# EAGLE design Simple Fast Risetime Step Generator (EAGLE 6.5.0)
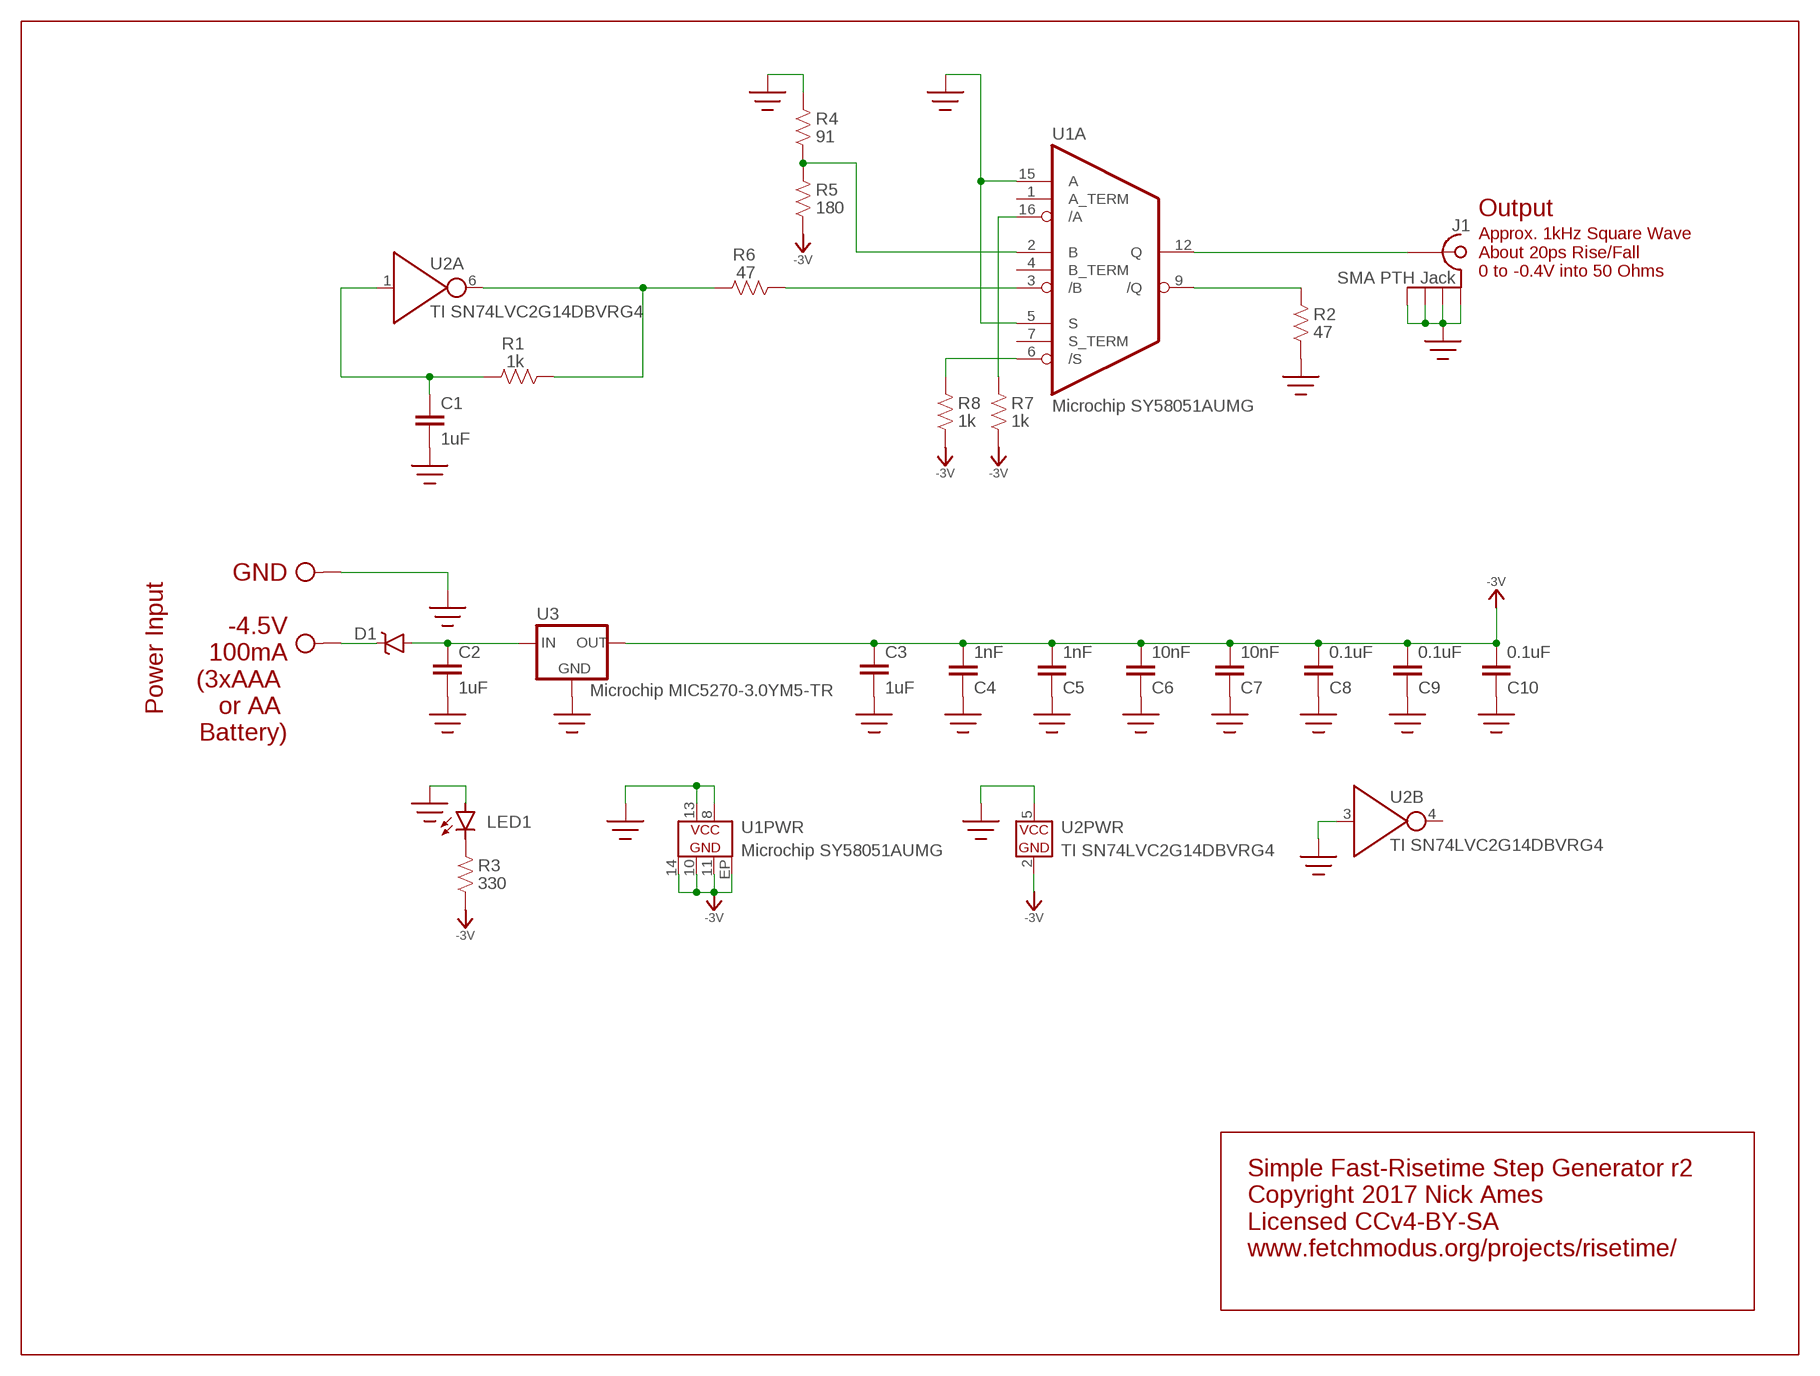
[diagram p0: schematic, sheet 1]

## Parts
C1  1uF  CAP402  [0402]
C2  1uF  CAP402  [0402]
C3  1uF  CAP402  [0402]
C4  1nF  CAP201  [0201]
C5  1nF  CAP201  [0201]
C6  10nF  CAP402  [0402]
C7  10nF  CAP402  [0402]
C8  0.1uF  CAP402  [0402]
C9  0.1uF  CAP402  [0402]
C10  0.1uF  CAP402  [0402]
D1  DIODE-SCHOTTKYSOD-523  [SOD-523]
J1  SMA PTH Jack  COAX-4GNDSMA-PTH  [CON-SMA-PTH]
LED1  LED0603  [LED-0603]
R1  1k  RESISTOR402  [0402@1]
R2  47  RESISTOR402  [0402@1]
R3  330  RESISTOR402  [0402@1]
R4  91  RESISTOR402  [0402@1]
R5  180  RESISTOR402  [0402@1]
R6  47  RESISTOR402  [0402@1]
R7  1k  RESISTOR402  [0402@1]
R8  1k  RESISTOR402  [0402@1]
TP1  TESTPOINTPTH  [TESTPOINT-1-PTH]
TP2  TESTPOINTPTH  [TESTPOINT-1-PTH]
U1  Microchip SY58051AUMG  SY58051AUMG  [QFN-16-3X3-MICREL]
U2  TI SN74LVC2G14DBVRG4  74LVC2G14  [SOT-23-6]
U3  Microchip MIC5270-3.0YM5-TR  V_REGSOT23-5-MIC5270  [SOT23-5]

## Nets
-3V: C3.1 C4.P$2 C5.P$2 C6.2 C7.2 C8.2 C9.2 C10.2 R3.1 R5.1 R7.1 R8.1 U1.10(PWR:V-) U1.11(PWR:V-1) U1.14(PWR:V-2) U1.EP(PWR:V-3) U2.2(PWR:V-) U3.4(OUT)
GND: C1.2 C2.2 C3.2 C4.P$1 C5.P$1 C6.1 C7.1 C8.1 C9.1 C10.1 J1.G1 J1.G2 J1.G3 J1.G4 LED1.A R2.1 R4.2 TP1.1 U1.5(A:S) U1.8(PWR:V+) U1.13(PWR:V+1) U1.15(A:A) U2.3(B:IN) U2.5(PWR:V+) U3.2(GND)
N$1: R6.1 U1.3(A:/B)
N$2: C1.1 R1.2 U2.1(A:IN)
N$3: R1.1 R6.2 U2.6(A:OUT)
N$4: D1.C TP2.1
N$5: R8.2 U1.6(A:/S)
N$6: C2.1 D1.A U3.5(IN)
N$7: J1.SIG(SIGNAL) U1.12(A:Q)
N$8: R2.2 U1.9(A:/Q)
N$9: LED1.C R3.2
N$10: R4.1 R5.2 U1.2(A:B)
N$13: R7.2 U1.16(A:/A)
Unconnected: U1.1(A:A_TERM) U1.4(A:B_TERM) U1.7(A:S_TERM) U2.4(B:OUT)

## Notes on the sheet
- Output
- Approx. 1kHz Square Wave
  About 20ps Rise/Fall
  0 to -0.4V into 50 Ohms
- GND
- -4.5V
  100mA
  (3xAAA 
  or AA 
  Battery)
- Power Input
- Simple Fast-Risetime Step Generator r2
  Copyright 2017 Nick Ames
  Licensed CCv4-BY-SA
  www.fetchmodus.org/projects/risetime/

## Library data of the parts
C1-C10 = NA-lib:CAP: Capacitor
D1 = NA-lib:DIODE-SCHOTTKY
J1 = NA-lib:COAX-4GND
LED1 = NA-lib:LED: LEDs
R1-R8 = NA-lib:RESISTOR: Resistor
TP1 TP2 = NA-lib:TESTPOINT
U1 = NA-lib:SY58051AUMG
U2 = NA-lib:74LVC2G14
U3 = NA-lib:V_REG

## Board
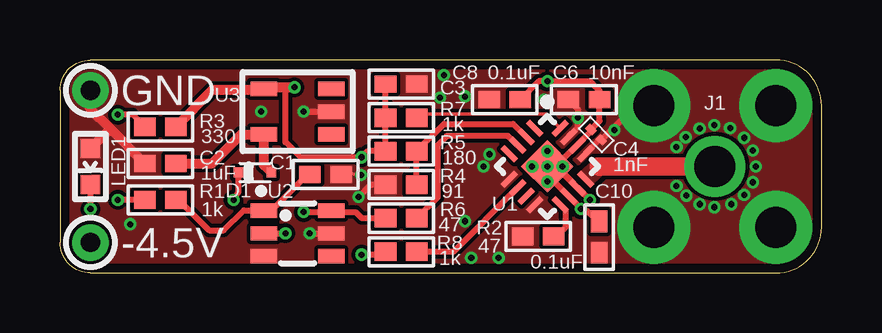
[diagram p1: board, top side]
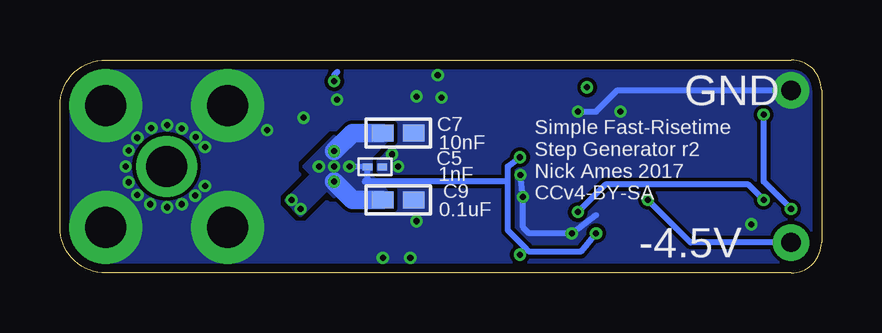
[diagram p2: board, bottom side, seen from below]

Size 31.75 x 8.89 mm. Coordinates in mm from the lower left corner, seen from the top.
Outline: 1.27,0 29.84,0 arc90 31.75,1.91 31.75,6.99 arc90 29.84,8.89 1.27,8.89 arc90 0,7.62 0,1.27 arc90 1.27,0
Copper layers (1*16): Top 0.0356mm / dielectric 1.5011mm / Bottom 0.0356mm
Design rules "LaenPCBOrder-tented_vias": minimum track width 6mil, minimum drill 10mil, track to track 6mil, track to pad 6mil, pad to pad 6mil, via to via 6mil, smd to smd 6mil, copper to edge 15mil, drill to drill 6mil, minimum pad ring 5mil, minimum via ring 5mil, stop-mask expansion 3mil, vias tented up to drill 25mil, thermal gap 10mil

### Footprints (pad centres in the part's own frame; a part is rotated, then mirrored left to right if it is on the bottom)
0402 = smd 0.9 x 0.7: 1 -0.65,0; 2 0.65,0
0201 = smd 0.406 x 0.279: P$1 -0.305,0; P$2 0.305,0
SOD-523 = smd 0.406 x 0.406: A 0.686,0; C -0.686,0
CON-SMA-PTH = drill 1.702 pad 3.048: G1 -2.54,2.54; G2 2.54,2.54; G3 -2.54,-2.54; G4 2.54,-2.54 | drill 1.702 pad 2.54: SIG 0,0
LED-0603 = smd 0.8 x 0.8: A -0.75,0; C 0.75,0
0402@1 = smd 0.9 x 0.762: 1 -0.65,0; 2 0.65,0
TESTPOINT-1-PTH = drill 0.8 pad 1.524: 1 0,0
QFN-16-3X3-MICREL = smd 0.8 x 0.23: 1 -1.5,0.75; 2 -1.5,0.25; 3 -1.5,-0.25; 4 -1.5,-0.75; 9 1.5,-0.75; 10 1.5,-0.25; 11 1.5,0.25; 12 1.5,0.75 | smd 0.23 x 0.8: 5 -0.75,-1.5; 6 -0.25,-1.5; 7 0.25,-1.5; 8 0.75,-1.5; 13 0.75,1.5; 14 0.25,1.5; 15 -0.25,1.5; 16 -0.75,1.5 | smd 1.55 x 1.55: EP 0,0
SOT-23-6 = smd 1.1 x 0.6: 1 -1.4,0.95; 2 -1.4,0; 3 -1.4,-0.95; 4 1.4,-0.95; 5 1.4,0; 6 1.4,0.95
SOT23-5 = smd 0.6 x 1.1: 1 -0.95,-1.4; 2 0,-1.4; 3 0.95,-1.4; 4 0.95,1.4; 5 -0.95,1.4

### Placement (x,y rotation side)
C1  11.07,4.11 0 top
C2  4.19,4.57 180 top
C3  14.22,7.87 0 top
C4  22.35,5.77 135 top
C5  18.62,4.42 180 bottom
C6  21.84,7.24 0 top
C7  17.65,5.84 180 bottom
C8  18.54,7.24 0 top
C9  17.65,3.05 180 bottom
C10  22.48,1.5 90 top
D1  8.13,4.19 0 top
J1  27.3,4.45 0 top
LED1  1.27,4.45 270 top
R1  4.19,3.05 0 top
R2  19.94,1.52 0 top
R3  4.19,6.1 180 top
R4  14.22,3.68 180 top
R5  14.22,5.08 0 top
R6  14.22,2.29 180 top
R7  14.22,6.48 0 top
R8  14.22,0.89 0 top
TP1  1.27,7.62 0 top
TP2  1.27,1.27 0 top
U1  20.32,4.45 315 top
U2  9.91,1.65 0 top
U3  9.91,6.73 90 top

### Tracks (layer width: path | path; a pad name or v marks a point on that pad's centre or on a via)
-3V  (via drill 0.25 pad 0.51)
  Top 0.254: 20.77,4.38 20.7,4.32 20.8,4.32 U1.11 21.59,3.56 v22.1,3.05 20.75,4.39 20.8,4.45 21.01,4.45 | 20.77,4.38 20.83,4.45 v20.95,4.45 | v20.32,3.81 20.32,4.06 20.35,4.06 U1.10 21.72,2.69 v21.72,2.67 21.86,2.67 C10.2 | 20.77,4.38 20.77,4.54 U1.14 22.14,5.91 C4.P$2 22.49,6.34 C6.2 22.49,7.61 22.1,8 v20.32,8 19.95,8 C8.2 | U2.2 v9.4,1.65 | 9.4,7.75 9.4,5.46 10.03,4.83 v12.57,4.83 12.83,5.08 R5.1 R7.1 C3.1 | R8.1 13.45,0.76 v12.57,0.76
  Top 0.406: R3.1 6.35,7.62 8.45,7.62 U3.4 8.57,7.75 9.4,7.75 v9.78,7.75
  Bottom 0.254: v19.68,4.45 C5.P$2 18.92,3.94 19.05,3.81 13.08,3.81 | v9.4,1.65 10.03,0.89 12.19,0.89 12.38,1.08 | 12.38,1.08 13.08,1.78 13.08,3.81 | 13.08,3.81 13.08,4.45 v12.57,4.83 | 20.19,8.38 20.32,8.26 v20.32,8 | v12.57,0.76 12.38,0.95 12.38,1.08
  Bottom 0.762: C7.2 19.56,5.84 v20.32,5.08 | C9.2 19.56,3.05 v20.32,3.81
  other vias: 20.32,4.45
  pour Bottom (no thermals): 19.05,4.45 20.32,5.71 21.59,4.45 20.32,3.17
  pour Bottom (no thermals): 20.68,3.43 21.72,2.39 22.35,3.02 21.29,4.09 20.75,3.56
  pour Bottom (no thermals): 18.72,4.09 18.72,4.83 18.08,5.46 19.43,5.46 19.74,5.16 19.74,3.73 19.43,3.43 18.08,3.43 18.08,3.45
GND  (via drill 0.25 pad 0.51)
  Top 0.152: C1.2 11.73,4.19 v12.55,4.09
  Top 0.254: U1.13 22.49,5.55 C4.P$1 24,6.99 J1.G1 | U1.15 21.59,6.07 v21.59,6.48 21.59,6.84 C6.1 | v10.16,6.73 U3.2 | v10.41,1.65 U2.5 | v12.45,3.17 12.95,3.68 R4.2
  Top 0.406: C2.2 2.09,6.03 | 2.09,6.03 1.27,6.84 TP1.1 | LED1.A 2.09,6.01 2.09,6.03
  Bottom 0.254: v12.55,4.09 v12.45,3.17 12.45,1.91 12.19,1.65 v10.41,1.65 9.4,2.41 | v10.16,6.73 9.4,6.73 8.51,7.62 TP1.1
  other vias: 2.92,2.03 8.38,6.73 16.89,7.37 16,8.26 20.19,7.24 17.91,4.95 17.65,4.45 18.29,0.64 17.14,0.64 16.89,2.16 27.28,6.17 29.01,4.45 27.28,2.74 26.11,3.23 26.67,2.87 27.99,2.87 28.52,3.25 28.88,3.78 28.88,5.11 28.52,5.64 27.94,6.05 26.67,6.02 26.09,5.66 25.7,5.26 25.7,3.63 23.11,5.97 15.85,7.32
  pour Bottom (isolate 0.152, rank 2, no thermals): 0,0 31.75,0 31.75,8.89 0,8.89
  pour Top (isolate 0.152, rank 2, no thermals): 0,0 31.75,0 31.75,8.89 0,8.89
N$1
  Top 0.254: U1.3 19.05,5.33 18.67,5.71 16.13,5.71 15.75,5.33 15.75,3.16 R6.1
N$2
  Top 0.254: C1.1 10.54,4.32 8.7,2.47 U2.1 | R1.2 4.95,3.05 6.22,1.78 6.83,1.78 7.67,2.62 8.49,2.62 U2.1 | 8.45,2.54 U2.1
N$3  (via drill 0.25 pad 0.51)
  Top 0.152: R1.1 3.56,3.05
  Top 0.254: 3.56,3.05 v2.41,3.05 | v10.16,2.54 11.24,2.54 U2.6 11.37,2.54 12.32,2.54 12.57,2.29 R6.2
  Bottom 0.254: v2.41,3.05 3.05,3.68 9.02,3.68 v10.16,2.54
N$4  (via drill 0.25 pad 0.51)
  Top 0.254: v7.24,3.05 7.44,3.38 D1.C
  Bottom 0.254: TP2.1 5.46,1.27 v7.24,3.05
N$5
  Top 0.254: U1.6 16.41,0.89 R8.2
N$6
  Top 0.406: D1.A 8.51,4.5 U3.5 7.56,5.78 6.35,4.57 C2.1
N$7
  Top 0.762: J1.SIG 22.48,4.45
  pour Top (no thermals): 21.56,4.11 22.3,4.83 22.99,4.83 22.99,4.06 22.61,4.06 22.12,3.58 22.1,3.58
N$8
  Top 0.254: U1.9 21.08,2.62 21.08,1.91 20.7,1.52 R2.2
N$9  (via drill 0.25 pad 0.51)
  Top 0.254: R3.2 3.03,6.6 v2.41,6.6 | LED1.C v1.27,2.67
  Bottom 0.254: v1.27,2.67 2.41,3.81 v2.41,6.6
N$10
  Top 0.254: R4.1 R5.2 16.02,6.22 18.9,6.22 U1.2
N$13
  Top 0.152: U1.16 20.28,6.63 15,6.63 R7.2

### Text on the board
tPlace: GND | -4.5V
bPlace: GND | Simple Fast-Risetime / Step Generator r2 / Nick Ames 2017 / CCv4-BY-SA | -4.5V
